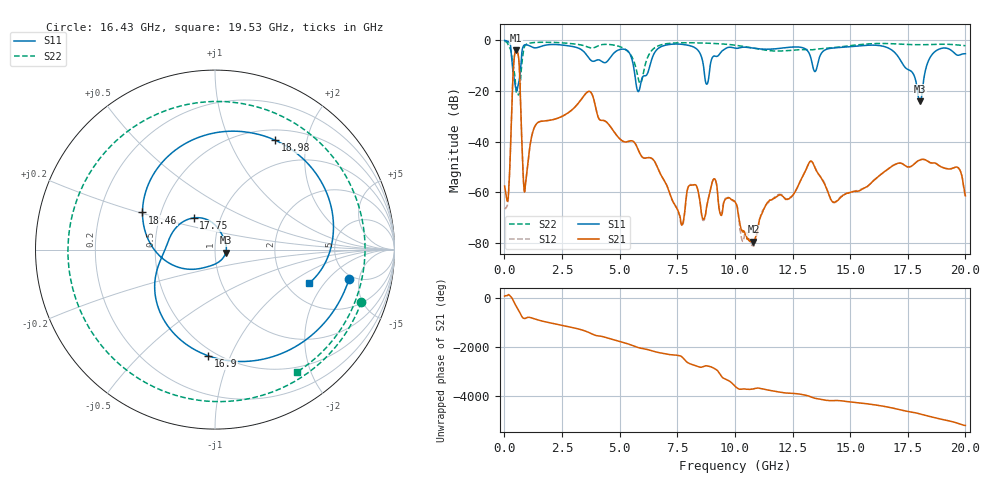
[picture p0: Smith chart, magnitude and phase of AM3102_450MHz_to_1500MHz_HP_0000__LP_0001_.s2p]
!Agilent Technologies,E8364B,MY43040894,A.07.50.67
!Agilent E8364B: A.07.50.67
!Date: Thursday, January 11, 2018 05:14:02
!Correction: S11(Full 2 Port(1,2))
!S21(Full 2 Port(1,2))
!S12(Full 2 Port(1,2))
!S22(Full 2 Port(1,2))
!S2P File: Measurements: S11, S21, S12, S22:
# Hz S  dB  R 50
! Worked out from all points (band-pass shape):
!   1601 points, 10 MHz to 20 GHz, reference 50 ohm
!   highest |S21| = -4.00 dB at 509.8 MHz (marker M1); lowest = -79.5 dB at 10.8 GHz (marker M2)
!   |S21| within 3 dB of the highest: 427.5 MHz to 618.8 MHz (191.2 MHz wide, 36.6 % of centre)
!   lowest |S11| = -24.1 dB at 18.03 GHz (marker M3), VSWR 1.13, Z = 56.3 - j1.95 ohm
!   |S11| at or under -10 dB: 346.8 MHz to 715.3 MHz (368.4 MHz wide, 69.4 % of centre); 5.597 GHz to 6.314 GHz (717.3 MHz wide, 12 % of centre); 17.33 GHz to 18.32 GHz (994.5 MHz wide, 5.58 % of centre)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
!   |S22| runs from -21.6 to -0.3 dB; largest |S21 - S12| = 0.0037
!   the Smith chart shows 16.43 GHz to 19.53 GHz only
!   S11 on the Smith chart (normalised r, x): 16.43 GHz: 4.59, -3.60; 16.9 GHz: 0.45, -0.83; 17.75 GHz: 0.74, +0.27; 18.46 GHz: 0.39, +0.21; 18.98 GHz: 0.64, +1.50; 19.53 GHz: 2.66, -1.43
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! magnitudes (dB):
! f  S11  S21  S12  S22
! 10 MHz  -0.1  -57.5  -66.3  -0.3
! 172.4 MHz  -0.6  -61.4  -62.2  -2.0
! 509.8 MHz  -18.5  -4.0  -4.0  -20.1
! 897.1 MHz  -1.8  -58.7  -58.3  -2.1
! 1.372 GHz  -3.0  -33.2  -33.2  -0.8
! 3.346 GHz  -3.7  -23.2  -23.2  -1.9
! 5.807 GHz  -20.3  -43.2  -43.3  -15.1
! 6.682 GHz  -3.2  -51.1  -51.1  -2.2
! 7.694 GHz  -1.6  -72.8  -73.1  -1.0
! 10.01 GHz  -3.1  -63.8  -63.6  -1.9
! 10.8 GHz  -3.1  -79.5  -80.8  -3.1
! 13.34 GHz  -8.7  -47.9  -47.9  -3.8
! 14.29 GHz  -3.0  -64.0  -64.1  -2.9
! 16.43 GHz  -2.3  -52.3  -52.3  -1.2
! 16.68 GHz  -3.1  -50.7  -50.5  -1.3
! 16.9 GHz  -4.5  -49.2  -49.2  -1.4
! 17.75 GHz  -13.4  -49.1  -49.0  -1.7
! 18.03 GHz  -24.1  -47.2  -47.2  -1.7
! 18.46 GHz  -6.9  -48.3  -48.3  -1.7
! 18.98 GHz  -3.2  -50.1  -50.1  -1.6
! 19.53 GHz  -5.1  -50.2  -50.2  -1.7
! 20 GHz  -5.3  -61.4  -62.4  -2.1
